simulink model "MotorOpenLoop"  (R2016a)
settings: Solver=VariableStepAuto  StartTime=0.0  StopTime=Tf  RelTol=1e-3
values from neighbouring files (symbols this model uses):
  d = 0    [Section4p2_DCMotorOpenLoop.m]    (also in Section4p3_DCMotorPControl.m; Section4p4_DCMotorPIControl.m; Section4p5_RocketPDControl.m = -0.01; Section4p6_PIDSecondOrder.m = 2)
  Gden = [1 a0]    [Section4p2_DCMotorOpenLoop.m]    (also in Section4p3_DCMotorPControl.m = [J*L (J*R+b*L) (Kt*Ke+b*R)]; Section4p4_DCMotorPIControl.m; Section4p5_RocketPDControl.m = [1 a1 a0]; Section4p6_PIDSecondOrder.m = [1 a1 a0])
  Gnum = b0    (= 766.8)    [Section4p2_DCMotorOpenLoop.m]    (also in Section4p3_DCMotorPControl.m = 0.00122680374957; Section4p4_DCMotorPIControl.m; Section4p5_RocketPDControl.m = 6.32; Section4p6_PIDSecondOrder.m = 17)
  Kol = 1/dcgain(G)    [Section4p2_DCMotorOpenLoop.m]
  r = 1000    [Section4p2_DCMotorOpenLoop.m]    (also in Section4p3_DCMotorPControl.m; Section4p4_DCMotorPIControl.m; Section4p5_RocketPDControl.m = 0.1; Section4p6_PIDSecondOrder.m = 4)
  Tf = 5    [Section4p2_DCMotorOpenLoop.m]    (also in Section4p3_DCMotorPControl.m = 0.005; Section4p4_DCMotorPIControl.m = 10; Section4p5_RocketPDControl.m = 10; Section4p6_PIDSecondOrder.m = 4)

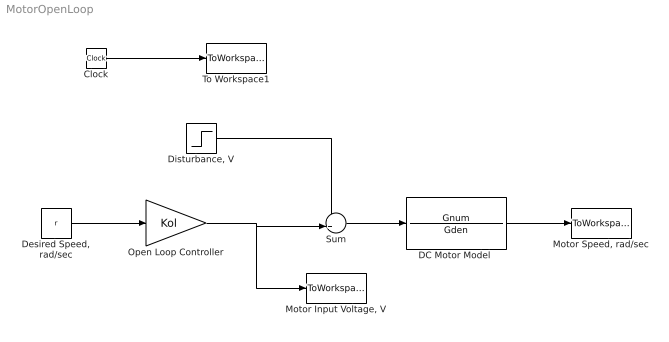
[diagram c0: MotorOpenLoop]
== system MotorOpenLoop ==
  Clock : Clock
  "DC Motor Model " : TransferFcn  Numerator=Gnum  Denominator=Gden
  "Desired Speed, rad/sec" : Constant  Value=r
  "Disturbance, V" : Step  Time=Tf/2  After=d  SampleTime=0
  "Motor Input Voltage, V" : ToWorkspace  VariableName=u  SampleTime=-1
  "Motor Speed, rad/sec" : ToWorkspace  VariableName=y  SampleTime=-1
  Open Loop Controller : Gain  Gain=Kol
  Sum : Sum  Inputs=++|
  To Workspace1 : ToWorkspace  VariableName=t  SampleTime=-1
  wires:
  Clock/1 -> To Workspace1/1
  "Disturbance, V"/1 -> Sum/1
  "Desired Speed, rad/sec"/1 -> Open Loop Controller/1
  Open Loop Controller/1 -> "Motor Input Voltage, V"/1, Sum/2
  Sum/1 -> "DC Motor Model "/1
  "DC Motor Model "/1 -> "Motor Speed, rad/sec"/1
